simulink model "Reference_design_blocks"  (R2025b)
settings: Solver=VariableStepAuto  StartTime=0.0  StopTime=10.0  RelTol=1e-3
InitFcn:
  | PreprocIndata = dataPreProc('data/sig_i.txt');
  | PreprocFirOutdata = dataPreProc('data/fir_o.txt');
  | PreprocFftOutdata = dataPreProc('data/fft_o.txt');
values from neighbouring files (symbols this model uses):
  tmp = reshape(sig_o_flt,Nfft,[])    [gen_vectors.m]
undefined symbols (not defined in the file or in its folder): code, Evaluation, fir_fft, FIR_FFT, fir_fft_ipconfig, netlist, None, Platform, S, VCK190, Versal, vmctmp, vsva2197, xcvc1902
libraries: matrix_library x6, dspsrcs4 x3, aieDSP x2, aieUtilities x2, aieBasic x1, vmcUtilities x1

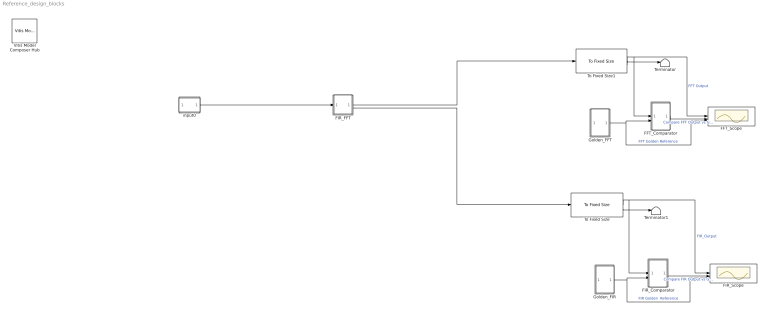
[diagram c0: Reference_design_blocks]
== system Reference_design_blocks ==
  FFT_Comparator : Subsystem
  FFT_Scope : Scope  NumInputPorts=3
  FIR_Comparator : Subsystem
  FIR_FFT : Subsystem
  FIR_Scope : Scope  NumInputPorts=3
  Golden_FFT : Subsystem
  Golden_FIR : Subsystem
  Terminator : Terminator
  Terminator1 : Terminator
  To Fixed Size : aieUtilities/To Fixed Size  Mode=Produce a valid output signal  OutputSize=2048  CopyMethod=Buffer samples to form output  HasStatusOutput=on
  To Fixed Size1 : aieUtilities/To Fixed Size  Mode=Produce a valid output signal  OutputSize=2048  CopyMethod=Buffer samples to form output  HasStatusOutput=on
  Vitis Model Composer Hub : vmcUtilities/Vitis Model Composer Hub  Tag=genX  CodeGeneration=off  SubsystemName=FIR_FFT  BlockHierPath=fir_fft/FIR_FFT  CompilationType=HDLCompilation  SubsystemType=AIENode  ExportTypeV2=IP Catalog  StartColumn=1  NumberOfColumns=1  TargetDirectory=./code  exportDesign=off  analyzeDesign=on  validateDesignOnHw=off  ExportType=AI Engines  IpVendor=xilinx.com  IpLibrary=hls  IpVersion=1.0  IpHWLanguage=Verilog  AieCompilerOptions={}  AieSimulatorOptions={}  CreateTestbench=on  TestbenchStackSize=10  RunRtlSim=off  RunCSim=off  RunAieSim=off  enableSimulationTimeout=on  enableGraphIterations=on  AieSimTimeout=50000  AieGraphIterations=-1  RunAieSimProfiling=off  LaunchVitisAnalyzer=off  PlotOutput=off  RunX86Sim=off  X86SimTimeout=10  GenHwImage=off  GenLibadfXo=off  GenHwValidationCode=off  PlatformType=Not Specified  HwSystemType=Baremetal  HwValidationTarget=hw  ProjDevice=Versal VCK190 Evaluation Platform (xcvc1902-vsva2197-2MP-e-S)  ProjDevicePart=xcvc1902-vsva2197-2MP-e-S  AIEType=AIE  SamplePeriod=-1  ClockFrequency=200  DataPathParallelism=1  xilinxfamily=versalaicore  part=xcvc1902  speed=-2MP-e-S  package=vsva2197  directory=./netlist  testbench=off  incr_netlist=off  synthesis_tool=Vivado  clock_wrapper=Clock Enables  dbl_ovrd=According to Block Masks  dcm_input_clock_period=10  sysclk_period=10  simulink_period=1  eval_field=0  IPInfoJsonString="{\"DUTSubsystemName\":\"FIR_FFT\",\"AIESubsystem\":{\"SubsystemName\":\"FIR_FFT\",\"TargetDirectory\":\"./code\",\"AIEArrayConfig\":\"Use entire AIE array\",\"StartColumn\":\"0\",\"NumberOfColumns\":\"1\"},\"SubsystemTag\":\"AIENode\"}"  LogFileName=/home/amd/training/vmc_filters/lab/code/model_composer.log  NThreads=4  IPConfigFile=/tmp/vmctmp-11086366910232838551/fir_fft_ipconfig.json
  input0 : Subsystem
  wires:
  To Fixed Size/1 -> FIR_Scope/1, FIR_Comparator/1(In1)  "FIR_Output"
  To Fixed Size/2 -> Terminator1/1
  FIR_Comparator/1(Out1) -> FIR_Scope/2  "Compare FIR Output vs Golden"
  Golden_FIR/1(Out1) -> FIR_Scope/3, FIR_Comparator/2(In2)  "FIR Golden  Reference"
  Golden_FFT/1(Out1) -> FFT_Scope/3, FFT_Comparator/2(In2)  "FFT Golden Reference"
  To Fixed Size1/1 -> FFT_Scope/1, FFT_Comparator/1(In1)  "FFT Output"
  FFT_Comparator/1(Out1) -> FFT_Scope/2  "Compare FFT Output vs Golden Reference"
  To Fixed Size1/2 -> Terminator/1
  input0/1(Out1) -> FIR_FFT/1(In1)
  FIR_FFT/1(Out1) -> To Fixed Size1/1
  FIR_FFT/2(Out2) -> To Fixed Size/1

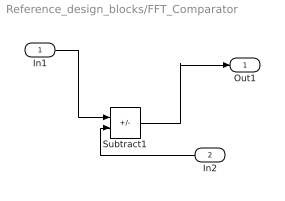
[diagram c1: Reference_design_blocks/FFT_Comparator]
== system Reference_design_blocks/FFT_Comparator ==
  In1 : Inport
  In2 : Inport  Port=2
  Subtract1 : Sum  Inputs=+-  OutDataTypeStr=double
  Out1 : Outport
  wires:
  In1/1 -> Subtract1/1
  In2/1 -> Subtract1/2
  Subtract1/1 -> Out1/1

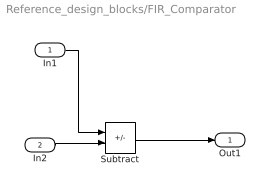
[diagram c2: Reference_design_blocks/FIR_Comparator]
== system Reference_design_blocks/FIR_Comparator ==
  In1 : Inport
  In2 : Inport  Port=2
  Subtract : Sum  Inputs=+-
  Out1 : Outport
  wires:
  Subtract/1 -> Out1/1
  In2/1 -> Subtract/2
  In1/1 -> Subtract/1

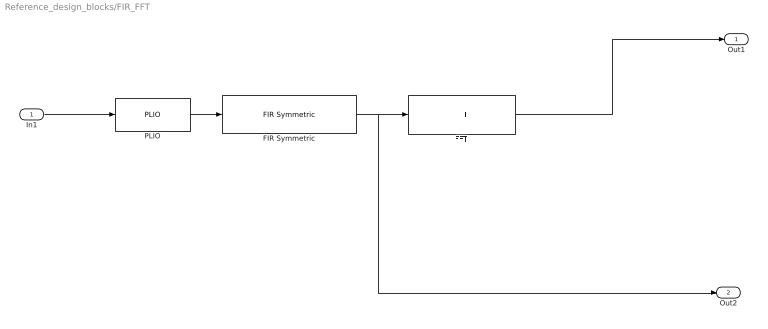
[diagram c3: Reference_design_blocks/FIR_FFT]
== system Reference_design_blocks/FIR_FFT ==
  In1 : Inport
  FFT : aieDSP/FFT  AIE_VARIANT=1  data_type=cint16  data_out_type=cint16  twiddle_type=cint16  point_size=256  input_window_size=2048  shift_val=6  rnd_mode=Round to positive infinity  sat_mode=0-None  ssr=1  twiddle_mode=0  use_ssr_widget_kernels=off  casc_length=1  transform_fft_nifft=1  TP_API=0  TP_DYN_PT_SIZE=0  blockJsonConstraints=[]  blockJsonConstraintsInternal=[]  spec=vmc_fft.json  SerializedMaskParamNames=[]  SerializedMaskParamValues=[]  SerializedMaskParamVisibilities=[]  block_type=FFT  SerializedMaskParamDataypes=uint|typename|typename|typename|uint|uint|uint|uint|uint|uint|uint|uint|uint|uint|uint|uint  SerializedMaskParamEnumStrArr=0|0|0|0|0|0|0|Round to positive infinity,Round to negative infinity,Round symmetrical to infinity,Round symmetrical to zero,Round convergent to even,Round convergent to odd|0-None,1-Asymmetric,3-Symmetric|0|0|0|0|0|0|0  SerializedMaskParamEnumValArr=0|0|0|0|0|0|0|2,3,4,5,6,7|0,1,3|0|0|0|0|0|0|0  SerializedMaskParamVectorArr=0|0|0|0|0|0|0|0|0|0|0|0|0|0|0|0  SerializedMaskParamKeys=AIE_VARIANT|TT_DATA|TT_OUT_DATA|TT_TWIDDLE|TP_POINT_SIZE|TP_WINDOW_VSIZE|TP_SHIFT|TP_RND|TP_SAT|TP_PARALLEL_POWER|TP_TWIDDLE_MODE|TP_USE_WIDGETS|TP_CASC_LEN|TP_FFT_NIFFT|TP_API|TP_DYN_PT_SIZE
  FIR Symmetric : aieDSP/FIR Symmetric  data_type=cint16  coef_type=int16  use_coeff_reload=off  dual_ip=off  num_outputs=off  coeff=[25 19 -108 78 181 -376 19 734 -804 -562 2147 -1224 -3491 9535 20445]  fir_length=29  input_window_size=2048  shift_val=15  rnd_mode=Round to positive infinity  sat_mode=0-None  casc_length=1  AIE_VARIANT=1  TP_API=0  ssr=1  blockJsonConstraints=[]  blockJsonConstraintsInternal=[]  spec=vmc_fir_sr_sym.json  SerializedMaskParamNames=[]  SerializedMaskParamValues=[]  SerializedMaskParamVisibilities=[]  block_type=FIR Symmetric  SerializedMaskParamDataypes=typename|typename|uint|uint|uint|coef_type|uint|uint|uint|uint|uint|uint|uint|uint|uint  SerializedMaskParamEnumStrArr=0|0|0|0|0|0|0|0|0|Floor,Ceiling,Round to positive infinity,Round to negative infinity,Round symmetrical to infinity,Round symmetrical to zero,Round convergent to even,Round convergent to odd|0-None,1-Asymmetric,3-Symmetric|0|0|0|0  SerializedMaskParamEnumValArr=0|0|0|0|0|0|0|0|0|0,1,2,3,4,5,6,7|0,1,3|0|0|0|0  SerializedMaskParamVectorArr=0|0|0|0|0|1|0|0|0|0|0|0|0|0|0  SerializedMaskParamKeys=TT_DATA|TT_COEFF|TP_USE_COEFF_RELOAD|TP_DUAL_IP|TP_NUM_OUTPUTS|coeff|TP_FIR_LEN|TP_INPUT_WINDOW_VSIZE|TP_SHIFT|TP_RND|TP_SAT|TP_CASC_LEN|AIE_VARIANT|TP_API|TP_SSR
  PLIO : aieBasic/PLIO  PlioWidth=64  PlioFreqSpec=off  PlioFreq=250  ColLocation=0  channel=0  blockJsonConstraints=[]  deprecateConstraints=0
  Out1 : Outport
  Out2 : Outport  Port=2
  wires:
  PLIO/1 -> FIR Symmetric/1
  In1/1 -> PLIO/1
  FFT/1 -> Out1/1
  FIR Symmetric/1 -> Out2/1, FFT/1

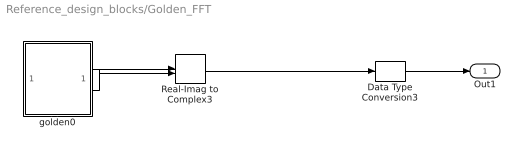
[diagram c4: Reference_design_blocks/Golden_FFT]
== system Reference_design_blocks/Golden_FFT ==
  Data Type Conversion3 : DataTypeConversion  OutDataTypeStr=int16
  Real-Imag to Complex3 : RealImagToComplex
  golden0 : Subsystem
  Out1 : Outport
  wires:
  Real-Imag to Complex3/1 -> Data Type Conversion3/1
  golden0/2(Out2) -> Real-Imag to Complex3/2
  golden0/1(Out1) -> Real-Imag to Complex3/1
  Data Type Conversion3/1 -> Out1/1

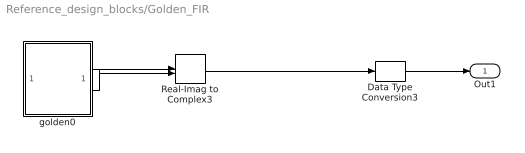
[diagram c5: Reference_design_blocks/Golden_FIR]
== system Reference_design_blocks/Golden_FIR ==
  Data Type Conversion3 : DataTypeConversion  OutDataTypeStr=int16
  Real-Imag to Complex3 : RealImagToComplex
  golden0 : Subsystem
  Out1 : Outport
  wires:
  Real-Imag to Complex3/1 -> Data Type Conversion3/1
  golden0/2(Out2) -> Real-Imag to Complex3/2
  golden0/1(Out1) -> Real-Imag to Complex3/1
  Data Type Conversion3/1 -> Out1/1

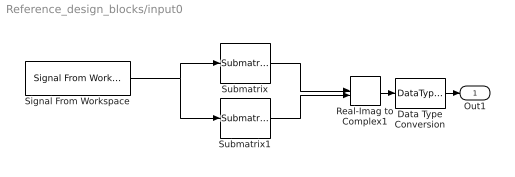
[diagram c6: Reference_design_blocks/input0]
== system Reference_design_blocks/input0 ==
  Data Type Conversion : DataTypeConversion  OutDataTypeStr=int16
  Real-Imag to Complex1 : RealImagToComplex
  Signal From Workspace : dspsrcs4/Signal From Workspace  X=PreprocIndata  Ts=1  nsamps=2048  OutputAfterFinalValue=Setting to zero  ignoreOrWarnInputAndFrameLengths=off  OutputFrames=off
  Submatrix : matrix_library/Submatrix  RowSpan=All rows  RowStartMode=First  RowStartIndex=1  RowEndMode=Last  RowEndIndex=1  ColSpan=One column  ColStartMode=First  ColStartIndex=1  ColEndMode=Last  ColEndIndex=1
  Submatrix1 : matrix_library/Submatrix  RowSpan=All rows  RowStartMode=First  RowStartIndex=1  RowEndMode=Last  RowEndIndex=1  ColSpan=One column  ColStartMode=Last  ColStartIndex=1  ColEndMode=Last  ColEndIndex=1
  Out1 : Outport
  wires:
  Signal From Workspace/1 -> Submatrix1/1, Submatrix/1
  Submatrix/1 -> Real-Imag to Complex1/1
  Submatrix1/1 -> Real-Imag to Complex1/2
  Real-Imag to Complex1/1 -> Data Type Conversion/1
  Data Type Conversion/1 -> Out1/1

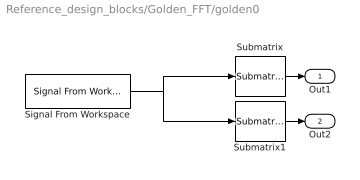
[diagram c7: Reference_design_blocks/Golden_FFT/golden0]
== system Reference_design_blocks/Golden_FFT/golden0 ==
  Signal From Workspace : dspsrcs4/Signal From Workspace  X=PreprocFftOutdata  Ts=1  nsamps=2048  OutputAfterFinalValue=Setting to zero  ignoreOrWarnInputAndFrameLengths=on  OutputFrames=off
  Submatrix : matrix_library/Submatrix  RowSpan=All rows  RowStartMode=First  RowStartIndex=1  RowEndMode=Last  RowEndIndex=1  ColSpan=One column  ColStartMode=First  ColStartIndex=1  ColEndMode=Last  ColEndIndex=1
  Submatrix1 : matrix_library/Submatrix  RowSpan=All rows  RowStartMode=First  RowStartIndex=1  RowEndMode=Last  RowEndIndex=1  ColSpan=One column  ColStartMode=Last  ColStartIndex=1  ColEndMode=Last  ColEndIndex=1
  Out1 : Outport  VectorParamsAs1DForOutWhenUnconnected=off
  Out2 : Outport  Port=2  VectorParamsAs1DForOutWhenUnconnected=off
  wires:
  Submatrix/1 -> Out1/1
  Signal From Workspace/1 -> Submatrix/1, Submatrix1/1
  Submatrix1/1 -> Out2/1

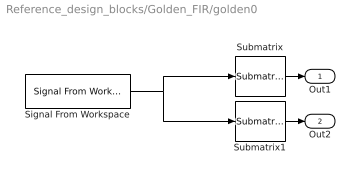
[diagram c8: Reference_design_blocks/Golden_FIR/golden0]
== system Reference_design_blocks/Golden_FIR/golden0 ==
  Signal From Workspace : dspsrcs4/Signal From Workspace  X=PreprocFirOutdata  Ts=1  nsamps=2048  OutputAfterFinalValue=Setting to zero  ignoreOrWarnInputAndFrameLengths=on  OutputFrames=off
  Submatrix : matrix_library/Submatrix  RowSpan=All rows  RowStartMode=First  RowStartIndex=1  RowEndMode=Last  RowEndIndex=1  ColSpan=One column  ColStartMode=First  ColStartIndex=1  ColEndMode=Last  ColEndIndex=1
  Submatrix1 : matrix_library/Submatrix  RowSpan=All rows  RowStartMode=First  RowStartIndex=1  RowEndMode=Last  RowEndIndex=1  ColSpan=One column  ColStartMode=Last  ColStartIndex=1  ColEndMode=Last  ColEndIndex=1
  Out1 : Outport  VectorParamsAs1DForOutWhenUnconnected=off
  Out2 : Outport  Port=2  VectorParamsAs1DForOutWhenUnconnected=off
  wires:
  Submatrix/1 -> Out1/1
  Signal From Workspace/1 -> Submatrix/1, Submatrix1/1
  Submatrix1/1 -> Out2/1
